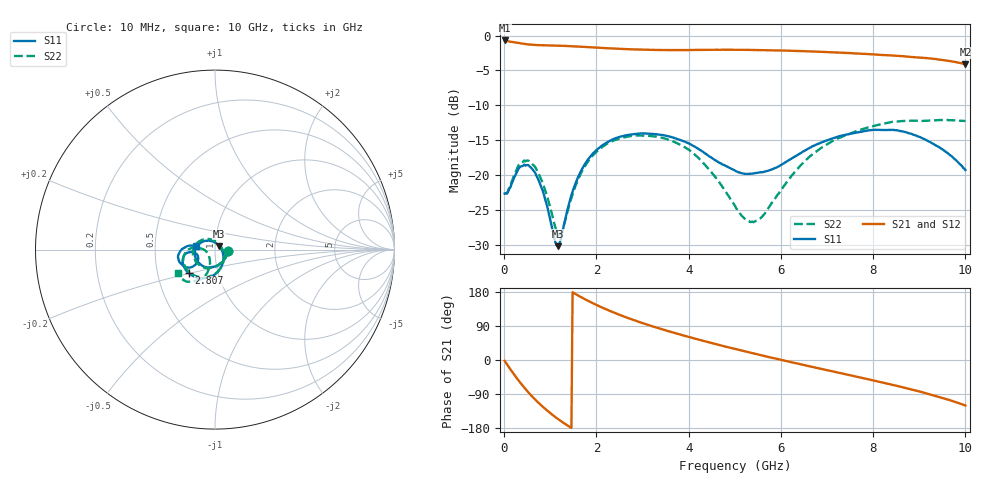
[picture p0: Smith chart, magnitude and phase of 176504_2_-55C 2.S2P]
!  2-Port S-parameters saved by WinCal
! VAR MeasName=S-Parameters (CALIBRATED_DATA) read from VNA (N5242A)
! VAR MeasDate=2017-11-2 17:07:49
! VAR NAME=176504_2_-55C 2
! VAR FILENAME=176504_2_-55C 2.S2P
! VAR DATE=2017-11-2 17:07:49
! VAR PHYS_PORTS=2,3
# Hz S DB R 50
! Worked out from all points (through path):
!   401 points, 10 MHz to 10 GHz, reference 50 ohm
!   highest |S21| = -0.70 dB at 10 MHz (marker M1); lowest = -4.1 dB at 10 GHz (marker M2)
!   lowest |S11| = -30.2 dB at 1.159 GHz (marker M3), VSWR 1.06, Z = 52.3 + j2.14 ohm
!   |S11| at or under -10 dB: start of sweep to end of sweep
!   |S22| runs from -28.6 to -12.1 dB; largest |S21 - S12| = 0.0085
!   S11 on the Smith chart (normalised r, x): 10 MHz: 1.16, -0.02; 2.807 GHz: 0.72, -0.20; 10 GHz: 0.81, +0.03
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1e7  -22.68 -5.4  -0.70 -2.1  -0.70 -2.1  -22.68 -5.6
1.34875e8  -21.80 -66.7  -0.89 -24.5  -0.89 -24.5  -21.59 -68.9
2.5975e8  -19.86 -105.0  -1.01 -45.5  -1.02 -45.6  -19.43 -107.2
4.84525e8  -18.60 -155.9  -1.24 -79.8  -1.25 -79.8  -17.96 -157.8
6.34375e8  -19.36 177.4  -1.33 -99.7  -1.33 -99.7  -18.60 175.5
8.34175e8  -22.21 142.6  -1.39 -123.1  -1.39 -123.0  -21.10 140.9
1.15885e9  -30.23 41.6  -1.45 -155.0  -1.44 -155.0  -28.42 52.4
1.25875e9  -28.39 -4.2  -1.47 -163.5  -1.47 -163.7  -27.98 9.0
1.45855e9  -22.92 -48.9  -1.53 -179.4  -1.53 -179.4  -23.31 -43.4
1.683325e9  -19.23 -74.1  -1.61 164.8  -1.61 164.8  -19.54 -71.9
2.2078e9  -15.43 -110.0  -1.81 133.9  -1.81 133.9  -15.63 -110.6
2.8072e9  -14.14 -137.8  -1.99 105.5  -2.00 105.5  -14.37 -140.6
3.35665e9  -14.23 -156.8  -2.07 83.5  -2.09 83.6  -14.60 -161.4
4.15585e9  -16.04 -173.3  -2.06 55.9  -2.07 56.0  -17.21 177.7
5.005e9  -19.39 -167.6  -2.04 29.1  -2.04 29.2  -24.45 -178.7
5.279725e9  -19.87 -160.5  -2.06 20.9  -2.06 21.1  -26.57 -157.8
5.529475e9  -19.65 -154.7  -2.09 13.6  -2.09 13.8  -26.31 -135.2
6.678325e9  -15.91 -143.0  -2.28 -18.1  -2.30 -18.1  -17.06 -108.7
7.577425e9  -14.02 -153.7  -2.56 -42.3  -2.58 -42.2  -13.88 -120.8
8.35165e9  -13.56 -167.3  -2.83 -63.6  -2.89 -63.5  -12.46 -131.5
9.25075e9  -15.35 176.4  -3.30 -91.2  -3.32 -90.8  -12.21 -140.5
1e10  -19.31 170.1  -4.12 -120.0  -4.13 -119.5  -12.27 -147.7
